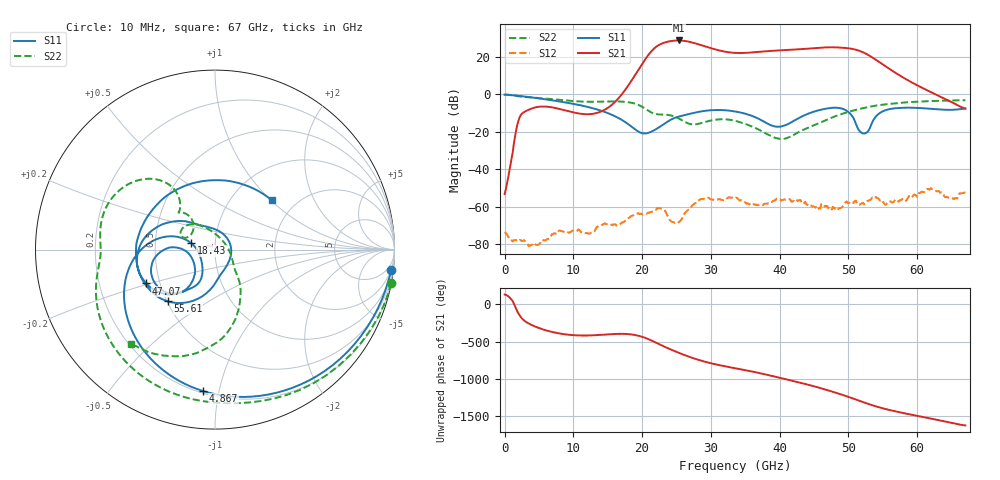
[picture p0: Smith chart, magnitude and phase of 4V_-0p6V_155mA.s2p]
! MARKI MICROWAVE INC.
! Date:  10/23/18
! Model Number:  AMM-6702CH
! Description:  2-port Small Signal S-parameter data for AMM-6702CH
! Frequency Range:  10 MHz to 67 GHz
! Port Configuration:  PORT 1: Input
!  PORT 2: Output
! Bias Condition: Vd = +4V, Vg = -0.6V
! AMM-6702CH s2p files are only valid for small signal conditions (below -5 dBm input power)
!S2P File: Measurements: Mag<S11> Ang<S11>, Mag<S21> Ang<S21>, Mag<S12> Ang<S12>, Mag<S22> Ang<S22>!row 1
# Hz S  dB  R 50
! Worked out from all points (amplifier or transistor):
!   401 points, 10 MHz to 67 GHz, reference 50 ohm
!   highest |S21| = 28.9 dB at 25.3 GHz (marker M1)
!   |S21| within 3 dB of that: 22.2 GHz to 29.01 GHz (6.813 GHz wide, 26.6 % of centre)
!   unconditionally stable (mu >= 1): start of sweep to end of sweep
!   at 11.06 GHz: K = 3305.09, MAG = -6.6 dB, |S12| = -73.4 dB
!   at 33.51 GHz: K = 19.75, MAG = 23.0 dB, |S12| = -55.7 dB
!   at 67 GHz: K = 213.32, MAG = -3.8 dB, |S12| = -52.6 dB
!   S11 on the Smith chart (normalised r, x): 10 MHz: 2, -17; 4.867 GHz: 0.21, -0.90; 18.43 GHz: 0.76, +0.06; 47.07 GHz: 0.42, -0.19; 55.61 GHz: 0.50, -0.34; 67 GHz: 1.51, +1.01
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1e7  -0.11 -6.7  -53.36 131.5  -73.74 172.3  -0.01 -10.8
4.866775e9  -2.04 -94.8  -6.64 47.3  -80.39 93.3  -1.87 -124.2
1.123082e10  -5.96 -165.5  -10.40 -58.0  -73.96 159.7  -3.81 -174.4
1.843225e10  -17.16 164.7  7.24 -43.4  -64.99 154.5  -4.44 141.8
2.0107e10  -20.80 -165.8  16.92 -78.2  -64.19 135.8  -6.85 125.8
2.127932e10  -20.03 -138.4  22.81 -121.2  -62.90 125.5  -9.52 125.9
2.245165e10  -17.61 -121.9  26.48 -173.3  -60.85 103.9  -10.71 133.3
2.362398e10  -14.75 -115.5  28.14 136.6  -64.43 66.1  -10.89 133.5
2.529872e10  -11.87 -122.1  28.89 71.4  -68.40 -123.6  -12.80 127.4
2.697348e10  -10.34 -128.4  28.07 12.6  -60.81 124.0  -15.82 139.1
2.898318e10  -8.83 -139.0  25.92 -45.4  -55.76 114.1  -14.91 158.6
3.3505e10  -9.10 -169.8  22.23 -136.0  -55.66 51.6  -14.09 134.9
3.702198e10  -13.16 176.8  22.81 159.3  -59.04 43.6  -18.91 105.3
4.0204e10  -17.14 -147.8  23.63 91.3  -56.84 35.3  -23.78 40.9
4.472582e10  -9.49 -132.1  24.73 -12.2  -59.92 53.7  -16.85 -42.2
4.707048e10  -7.40 -153.7  25.21 -74.2  -60.76 -41.5  -13.19 -52.3
4.857775e10  -7.22 -174.8  25.12 -117.4  -61.01 -47.0  -11.00 -59.7
5.041998e10  -10.98 146.4  24.45 -174.3  -58.50 166.0  -8.89 -68.6
5.242968e10  -20.80 -3.6  22.01 119.0  -57.93 -114.2  -7.09 -78.4
5.56117e10  -8.16 -132.5  14.51 31.1  -58.20 93.0  -5.22 -94.2
5.594665e10  -7.85 -137.2  13.70 23.6  -57.06 16.7  -5.09 -95.6
6.7e10  -7.56 41.3  -7.56 175.9  -52.63 22.5  -3.07 -131.6
